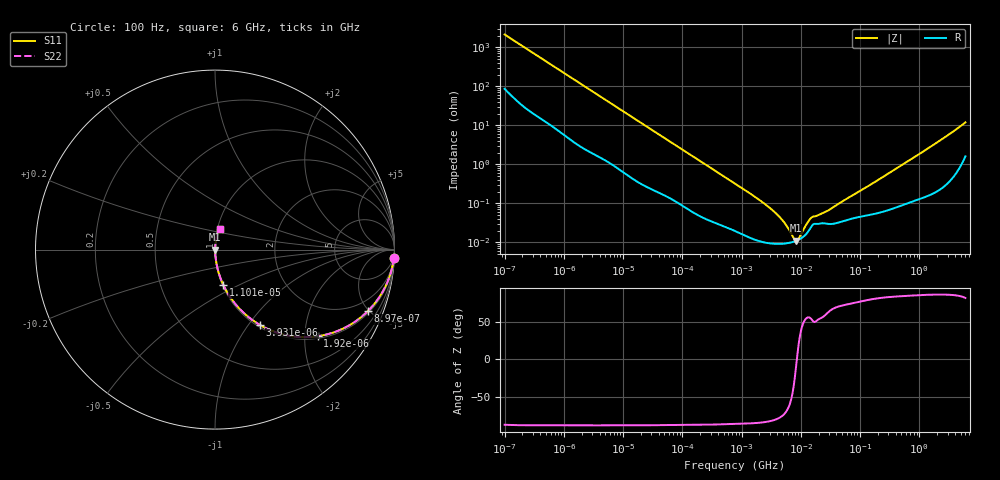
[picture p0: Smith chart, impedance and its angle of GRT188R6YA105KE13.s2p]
!Murata Part Number: GRT188R6YA105KE13
!These Parameters are Measured in Series Mode Connection
!Data Generated on Jun 19, 2026
!  o--ll--o
!Port1  Port2
!  o------o
!Operation Temp=25[degC], DC Bias Voltage=0[V]
!Freq. Start=100[Hz] Stop=6[GHz] 401[Steps]
# Hz S RI R 50
!Freq.(Hz) S11(Real) S11(Imag) S21(Real) S21(Imag) S12(Real) S12(Imag) S22(Real) S22(Imag)
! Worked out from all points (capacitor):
!   401 points, 100 Hz to 6 GHz, reference 50 ohm
!   read as one part in series: C = 742 nF near 109 Hz
!   lowest |Z| = 11 mohm at 8.312 MHz (marker M1)
!   series resonance near 8.573 MHz, so ESL is about 460 pH
!   S11 on the Smith chart (normalised r, x): 100 Hz: 3, -43; 897 Hz: 1.13, -4.91; 1.92 kHz: 1.06, -2.32; 3.931 kHz: 1.03, -1.14; 11.01 kHz: 1.01, -0.42; 6 GHz: 1.03, +0.23
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100  0.9959 -0.0465  0.00406 0.0465  0.00406 0.0465  0.9959 -0.0465
335  0.9727 -0.1497  0.0273 0.1497  0.0273 0.1497  0.9727 -0.1497
897  0.8513 -0.3429  0.1487 0.3429  0.1487 0.3429  0.8513 -0.3429
1920  0.5714 -0.4828  0.4286 0.4828  0.4286 0.4828  0.5714 -0.4828
2008  0.5502 -0.4854  0.4498 0.4854  0.4498 0.4854  0.5502 -0.4854
3931  0.2523 -0.4211  0.7477 0.4211  0.7477 0.4211  0.2523 -0.4211
6433  0.1176 -0.3083  0.8824 0.3083  0.8824 0.3083  0.1176 -0.3083
11009  0.0465 -0.1975  0.9535 0.1975  0.9535 0.1975  0.0465 -0.1975
40335  0.00519 -0.0576  0.9948 0.0576  0.9948 0.0576  0.00519 -0.0576
774597  0.000205 -0.00321  0.9998 0.00321  0.9998 0.00321  0.000205 -0.00321
1983483  0.000109 -0.00122  0.9999 0.00122  0.9999 0.00122  0.000109 -0.00122
3549919  9.18e-05 -0.000602  0.9999 0.000602  0.9999 0.000602  9.18e-05 -0.000602
5079039  9.21e-05 -0.000331  0.9999 0.000331  0.9999 0.000331  9.21e-05 -0.000331
7599586  0.000104 -7.35e-05  0.9999 7.35e-05  0.9999 7.35e-05  0.000104 -7.35e-05
8311524  0.000109 -1.88e-05  0.9999 1.88e-05  0.9999 1.88e-05  0.000109 -1.88e-05
9090158  0.000116 3.61e-05  0.9999 -3.61e-05  0.9999 -3.61e-05  0.000116 3.61e-05
1.300572e7  0.000179 0.000266  0.9998 -0.000266  0.9998 -0.000266  0.000179 0.000266
1.555665e7  0.000271 0.000352  0.9997 -0.000352  0.9997 -0.000352  0.000271 0.000352
2.911731e7  0.000296 0.000585  0.9997 -0.000585  0.9997 -0.000585  0.000296 0.000585
3.124326e8  0.000715 0.00597  0.9993 -0.00597  0.9993 -0.00597  0.000715 0.00597
1.95892e9  0.00324 0.0354  0.9968 -0.0354  0.9968 -0.0354  0.00324 0.0354
6e9  0.0287 0.1123  0.9713 -0.1123  0.9713 -0.1123  0.0287 0.1123
